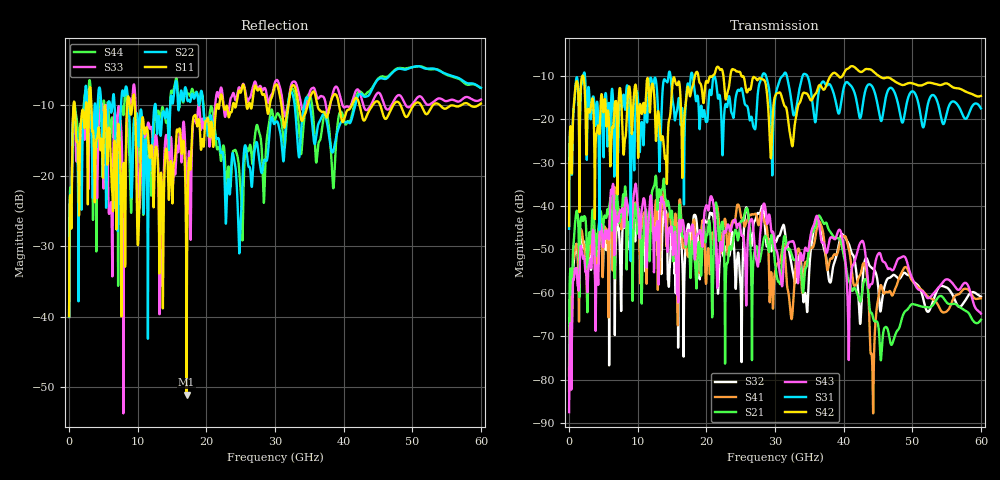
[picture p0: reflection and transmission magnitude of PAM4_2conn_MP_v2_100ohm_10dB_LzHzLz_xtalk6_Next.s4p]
! Info: Touchstone file created by Circ.  Input file=FAB50GbE_2conn_Midplane_Examax_Topo2_v2_100ohm_10dB_LzHzLz.circ
# Hz S RI R 50
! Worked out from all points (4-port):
!   6000 points, 10 MHz to 60 GHz, reference 50 ohm
!   strongest paths, dB at 10 MHz, 15.01 GHz, 30.01 GHz, 45.01 GHz, 60 GHz:
!     S42: -44.7, -13.0, -14.7, -9.9, -14.7
!     S31: -45.3, -14.5, -15.5, -17.1, -17.5
!     S43: -87.5, -46.2, -49.3, -51.1, -64.8
!     S21: -77.7, -41.6, -53.3, -67.2, -66.2
!     S41: -82.6, -46.1, -55.2, -61.7, -61.3
!     S32: -79.1, -43.9, -48.2, -58.2, -60.9
!   lowest |S11| = -51.1 dB at 17.13 GHz (marker M1), VSWR 1.01, Z = 50.3 - j0.118 ohm
!   |S11| at or under -10 dB: 3.236 GHz to 8.459 GHz (5.224 GHz wide, 89.3 % of centre); 9.59 GHz to 21.52 GHz (11.93 GHz wide, 76.7 % of centre); 42.34 GHz to 44.2 GHz (1.867 GHz wide, 4.31 % of centre)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
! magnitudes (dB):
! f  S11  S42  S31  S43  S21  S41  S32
! 10 MHz  -40.0  -44.7  -45.3  -87.5  -77.7  -82.6  -79.1
! 1.98 GHz  -10.6  -10.0  -11.4  -51.5  -43.3  -47.4  -48.5
! 6.23 GHz  -21.6  -23.4  -13.2  -37.1  -45.5  -41.7  -40.2
! 17.13 GHz  -51.1  -14.1  -13.7  -47.9  -47.8  -49.8  -46.4
! 24.85 GHz  -8.0  -9.1  -13.5  -44.1  -45.2  -40.6  -55.1
! 44.17 GHz  -10.1  -8.8  -12.5  -57.9  -64.9  -76.3  -54.3
! 60 GHz  -9.7  -14.7  -17.5  -64.8  -66.2  -61.3  -60.9
